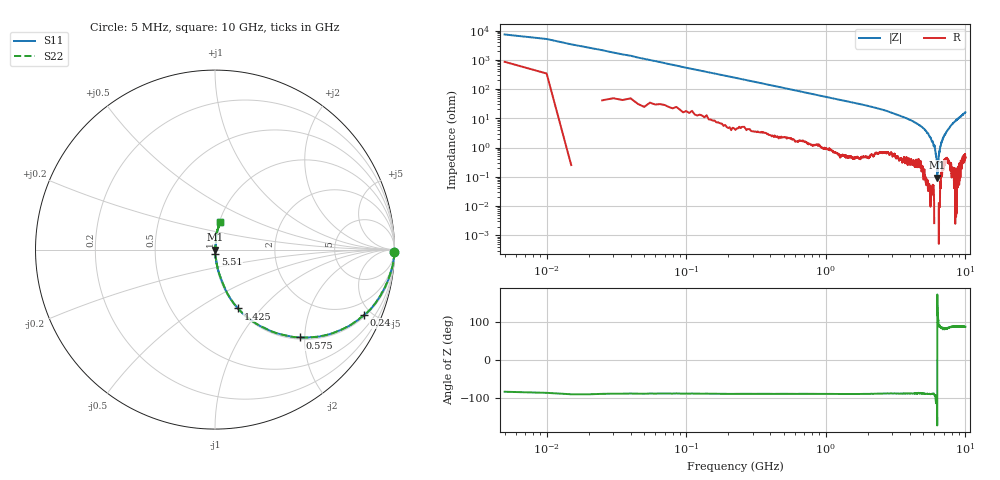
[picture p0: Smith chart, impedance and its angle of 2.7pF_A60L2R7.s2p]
! Amotech Co.,Ltd.
! http://www.amotech.co.kr/
! Part Number: A60L2R7
! These Parameters are Measured in Series Mode Connection
! Operation Temp=25[degC], DC Bias Voltage=0[V]
! Freq. Start=5[MHz] Stop=10[GHz], 2000[Steps]
! Date: Monday, July 14, 2020, 09:29:59
# GHZ S RI R 50.000000
!Freq.(Hz) S11(Real) S11(Imag) S21(Real) S21(Imag) S12(Real) S12(Imag) S22(Real) S22(Imag)
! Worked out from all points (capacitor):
!   2000 points, 5 MHz to 10 GHz, reference 50 ohm
!   read as one part in series: C = 2.97 pF near 55 MHz
!   lowest |Z| = 94.6 mohm at 6.285 GHz (marker M1)
!   series resonance near 6.288 GHz, so ESL is about 220 pH
!   S11 on the Smith chart (normalised r, x): 5 MHz: open; 240 MHz: 1.10, -4.52; 575 MHz: 1.04, -1.89; 1.425 GHz: 1.01, -0.76; 5.51 GHz: 1.00, -0.05; 10 GHz: 1.01, +0.32
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0.005  0.9982 -0.0135  0.00177 0.0135  0.00177 0.0135  0.9982 -0.0135
0.065  0.9817 -0.117  0.0183 0.117  0.0183 0.117  0.9817 -0.117
0.095  0.9647 -0.1709  0.0353 0.1709  0.0353 0.1709  0.9647 -0.1709
0.155  0.9184 -0.262  0.0816 0.262  0.0816 0.262  0.9184 -0.262
0.24  0.8309 -0.3636  0.1691 0.3636  0.1691 0.3636  0.8309 -0.3636
0.575  0.4722 -0.4895  0.5278 0.4895  0.5278 0.4895  0.4722 -0.4895
0.945  0.2501 -0.4245  0.7499 0.4245  0.7499 0.4245  0.2501 -0.4245
1.425  0.1283 -0.3279  0.8717 0.3279  0.8717 0.3279  0.1283 -0.3279
1.675  0.097 -0.2886  0.903 0.2886  0.903 0.2886  0.097 -0.2886
3.34  0.0192 -0.1224  0.9808 0.1224  0.9808 0.1224  0.0192 -0.1224
5.005  0.00305 -0.0451  0.9969 0.0451  0.9969 0.0451  0.00305 -0.0451
5.51  0.00114 -0.0247  0.9989 0.0247  0.9989 0.0247  0.00114 -0.0247
6.035  -0.000597 -0.0108  1.001 0.0108  1.001 0.0108  -0.000597 -0.0108
6.19  -0.00179 -0.0044  1.002 0.0044  1.002 0.0044  -0.00179 -0.0044
6.285  -0.000938 -0.000127  1.001 0.000127  1.001 0.000127  -0.000938 -0.000127
6.325  -0.000981 0.000987  1.001 -0.000987  1.001 -0.000987  -0.000981 0.000987
6.495  -9.6e-05 0.0067  1 -0.0067  1 -0.0067  -9.6e-05 0.0067
6.67  0.000897 0.0121  0.9991 -0.0121  0.9991 -0.0121  0.000897 0.0121
6.9  0.00323 0.0202  0.9968 -0.0202  0.9968 -0.0202  0.00323 0.0202
7.275  0.00461 0.0327  0.9954 -0.0327  0.9954 -0.0327  0.00461 0.0327
8.335  0.00628 0.074  0.9937 -0.074  0.9937 -0.074  0.00628 0.074
10  0.0296 0.1561  0.9704 -0.1561  0.9704 -0.1561  0.0296 0.1561
